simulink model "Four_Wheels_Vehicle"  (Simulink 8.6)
settings: Solver=ode45  StartTime=0.0  StopTime=20  RelTol=1e-3
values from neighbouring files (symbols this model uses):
  beta = 1    [Vehicle_Parameters.m]
  g = 9.81    [Vehicle_Parameters.m]
  H_CoG = 0.700    (= 0.7)    [Vehicle_Parameters.m]
  Hearo = 0.750    (= 0.75)    [Vehicle_Parameters.m]
  Iz = 2480    [Vehicle_Parameters.m]
  Jw = 2.166    [Vehicle_Parameters.m]
  L = 10    [Vehicle_Parameters.m]
  Lf = 1.180    (= 1.18)    [Vehicle_Parameters.m]
  Lr = 1.770    (= 1.77)    [Vehicle_Parameters.m]
  Lw = 1.880    (= 1.88)    [Vehicle_Parameters.m]
  m = 1500    [Vehicle_Parameters.m]
  miu = 0.85    [Vehicle_Parameters.m]
  reff = 0.380    (= 0.38)    [Vehicle_Parameters.m]
undefined symbols (not defined in the file or in its folder): DiscIntNeverNeededParam, Init, Ki, Kp, LowerLimit, sigbuilder_block, Ts, UpperLimit
libraries: simulink x15, powerlib_extras x3
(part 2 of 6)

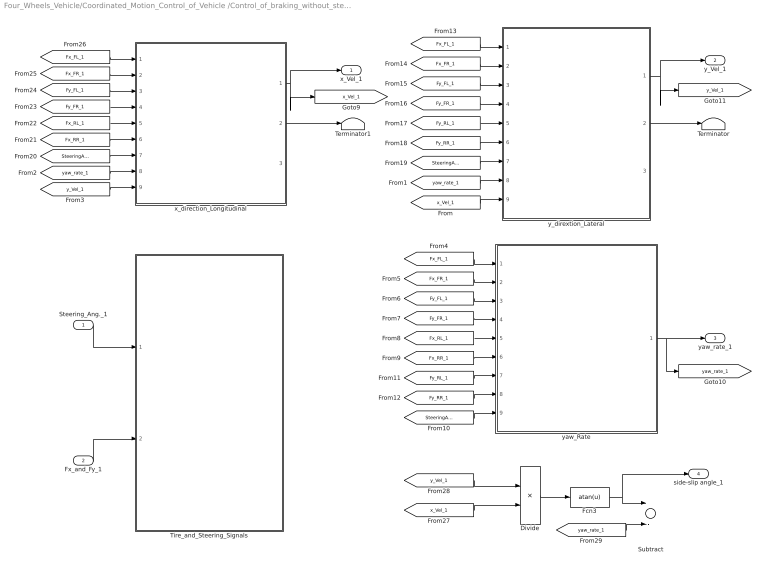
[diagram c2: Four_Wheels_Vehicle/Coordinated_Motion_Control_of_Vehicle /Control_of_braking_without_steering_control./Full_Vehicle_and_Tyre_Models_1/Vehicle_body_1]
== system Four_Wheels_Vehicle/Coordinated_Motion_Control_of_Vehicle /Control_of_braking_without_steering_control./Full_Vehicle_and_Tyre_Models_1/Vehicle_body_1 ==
  Steering_Ang._1 : Inport
  Fx_and_Fy_1 : Inport  Port=2
  Divide : Product  Inputs=*/
  Fcn3 : Fcn  Expr=atan(u)
  Subtract : Sum  Inputs=+-
  Terminator : Terminator
  Terminator1 : Terminator
  Tire_and_Steering_Signals : Subsystem
  x_direction_Longitudinal : Subsystem
  y_dirextion_Lateral : Subsystem
  yaw_Rate : Subsystem
  x_Vel_1 : Outport
  y_Vel_1 : Outport  Port=2
  yaw_rate_1 : Outport  Port=3
  side-slip angle_1 : Outport  Port=4
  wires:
  Fx_and_Fy_1/1 -> Tire_and_Steering_Signals/2(Fx_and_Fy)
  [yaw_rate_1] -> Subtract/2
  [y_Vel_1] -> Divide/1
  [x_Vel_1] -> Divide/2
  Fcn3/1 -> Subtract/1, side-slip angle_1/1
  Divide/1 -> Fcn3/1
  Steering_Ang._1/1 -> Tire_and_Steering_Signals/1(Steering_Ang.)
  yaw_Rate/1(yaw_rate_1) -> yaw_rate_1/1, [yaw_rate_1]
  [Fx_FL_1] -> x_direction_Longitudinal/1(Fx_FL_1)
  [Fx_FR_1] -> x_direction_Longitudinal/2(Fx_FR_1)
  [Fy_FL_1] -> x_direction_Longitudinal/3(Fy_FL_1)
  [Fy_FR_1] -> x_direction_Longitudinal/4(Fy_FR_1)
  [Fx_RL_1] -> x_direction_Longitudinal/5(Fx_RL_1)
  [Fx_RR_1] -> x_direction_Longitudinal/6(Fx_RR_1)
  [SteeringAng_1] -> x_direction_Longitudinal/7(Steering_Ang_1)
  [SteeringAng_1] -> y_dirextion_Lateral/7(Steering_Ang._1)
  [Fy_RR_1] -> y_dirextion_Lateral/6(Fy_RR_1)
  [Fy_RL_1] -> y_dirextion_Lateral/5(Fy_RL_1)
  [Fy_FR_1] -> y_dirextion_Lateral/4(Fy_FR_1)
  [Fy_FL_1] -> y_dirextion_Lateral/3(Fy_FL_1)
  [Fx_FR_1] -> y_dirextion_Lateral/2(Fx_FR_1)
  [Fx_FL_1] -> y_dirextion_Lateral/1(Fx_FL_1)
  [SteeringAng_1] -> yaw_Rate/9(Steering_Ang._1)
  [Fy_RR_1] -> yaw_Rate/8(Fy_RR_1)
  [Fy_RL_1] -> yaw_Rate/7(Fy_RL_1)
  [Fx_RR_1] -> yaw_Rate/6(Fx_RR_1)
  [Fx_RL_1] -> yaw_Rate/5(Fx_RL_1)
  [Fy_FR_1] -> yaw_Rate/4(Fy_FR_1)
  [Fy_FL_1] -> yaw_Rate/3(Fy_FL_1)
  [Fx_FR_1] -> yaw_Rate/2(Fx_FR_1)
  [Fx_FL_1] -> yaw_Rate/1(Fx_FL_1)
  [y_Vel_1] -> x_direction_Longitudinal/9(y_Vel_1)
  y_dirextion_Lateral/1(y_Vel_1) -> y_Vel_1/1, [y_Vel_1]
  [yaw_rate_1] -> x_direction_Longitudinal/8(yaw_rate_1)
  [yaw_rate_1] -> y_dirextion_Lateral/8(yaw_rate_1)
  [x_Vel_1] -> y_dirextion_Lateral/9(x_Vel_1)
  x_direction_Longitudinal/1(x_Vel_1) -> x_Vel_1/1, [x_Vel_1]
  x_direction_Longitudinal/2(x total force) -> Terminator1/1
  y_dirextion_Lateral/2(y total force) -> Terminator/1

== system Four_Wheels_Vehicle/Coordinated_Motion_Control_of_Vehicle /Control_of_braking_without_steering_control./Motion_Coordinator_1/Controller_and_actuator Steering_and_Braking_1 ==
  StteringAng : Inport
  Reference_Steering : Inport  Port=2
  Reference_Sideslip : Inport  Port=3
  Feedback_Steering : Inport  Port=4
  Feedback_Sideslip : Inport  Port=5
  Brake_controller_1 : Subsystem
  Brake_controller_2 : Subsystem
  Brake_controller_3 : Subsystem
  Brake_controller_4 : Subsystem
  Steering_controller : Subsystem
  f : Outport
  Mzc_1 : Outport  Port=2
  Mzc_2 : Outport  Port=3
  Mzc_3 : Outport  Port=4
  Mzc_4 : Outport  Port=5
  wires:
  Brake_controller_4/1(Mzc_4) -> Mzc_4/1
  Brake_controller_3/1(Mzc_3) -> Mzc_3/1
  Brake_controller_2/1(Mzc_2) -> Mzc_2/1
  Brake_controller_1/1(Mzc_1) -> Mzc_1/1
  Feedback_Sideslip/1 -> Brake_controller_1/2(Feedback_Sideslip_1), Brake_controller_2/2(Feedback_Sideslip_2), Brake_controller_3/2(Feedback_Sideslip_3), Brake_controller_4/2(Feedback_Sideslip_4)
  Reference_Sideslip/1 -> Brake_controller_1/1(Reference_Sideslip_1), Brake_controller_2/1(Reference_Sideslip_2), Brake_controller_3/1(Reference_Sideslip_3), Brake_controller_4/1(Reference_Sideslip_4)
  Steering_controller/1(f) -> f/1
  Feedback_Steering/1 -> Steering_controller/3(Feedback_Steering)
  Reference_Steering/1 -> Steering_controller/2(Reference_Steering)
  StteringAng/1 -> Steering_controller/1(StteringAng)

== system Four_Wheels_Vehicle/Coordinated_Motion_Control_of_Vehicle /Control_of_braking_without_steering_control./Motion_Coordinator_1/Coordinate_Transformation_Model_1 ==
  note: vehicle heading
  delta_steer (rad) : Inport
  v_x (m/s) : Inport  Port=2
  1/L : Gain  Gain=1/L
  Beta : Scope
  Beta1 : Scope
  Divide : Product  Inputs=*/
  Gain : Gain  Gain=L/2
  Gain1 : Gain  Gain=0.1
  Gain2 : Gain  Gain=0.1
  Gain4 : Gain  Gain=0.345
  Ground : Ground
  Integrator : Integrator
  Integrator1 : Integrator  LimitOutput=on  UpperSaturationLimit=0
  Integrator2 : Integrator
  Product{,1,3..4} (4 alike) : Product
  Sideslip_angle : Scope
  Subtract : Sum  Inputs=+-
  Sum : Sum  Inputs=|+-
  Sum1 : Sum  Inputs=|++
  Terminator : Terminator
  Trigonometric Function : Trigonometry  Operator=cos
  Trigonometric Function1 : Trigonometry
  Trigonometric Function2 : Trigonometry  Operator=atan
  Trigonometric Function3 : Trigonometry  Operator=tan
  steerVsYawrate1 : Scope  NumInputPorts=3
  steerVsYawrate2 : Scope  NumInputPorts=3
  yaw_rate : Product
  X-position : Outport
  Y-position : Outport  Port=2
  yaw_Rate : Outport  Port=3
  Sideslip_beta : Outport  Port=4
  yaw_pos. : Outport  Port=5
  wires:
  Subtract/1 -> Beta/1
  Gain4/1 -> Divide/1, Integrator1/1, steerVsYawrate2/3
  Trigonometric Function2/1 -> Subtract/1, Sideslip_beta/1, Sideslip_angle/1
  Gain2/1 -> Integrator2/1
  Gain1/1 -> Trigonometric Function1/1, yaw_pos./1, steerVsYawrate1/3, Trigonometric Function/1
  delta_steer (rad)/1 -> yaw_rate/2
  Divide/1 -> Trigonometric Function2/1
  Trigonometric Function3/1 -> Terminator/1
  Ground/1 -> Trigonometric Function3/1
  Product4/1 -> Sum1/2
  Product3/1 -> Sum/2
  Gain/1 -> Product4/1, Product3/1  "L/2*psi-dot"
  Sum1/1 -> Gain4/1  "v_Y (m/s)"
  Sum/1 -> Divide/2, Integrator/1, steerVsYawrate2/2  "v_X (m/s)"
  1/L/1 -> yaw_rate/1  "v_x / L"
  yaw_rate/1 -> Gain2/1, yaw_Rate/1, Subtract/2, Beta1/1, Gain/1, steerVsYawrate2/1
  v_x (m/s)/1 -> 1/L/1, Product1/1, Product/1  "v_x (m/s)"
  Integrator1/1 -> Y-position/1, steerVsYawrate1/2
  Integrator/1 -> X-position/1, steerVsYawrate1/1
  Integrator2/1 -> Gain1/1  "yaw_heading (rad)"
  Trigonometric Function1/1 -> Product3/2, Product/2  "sin(psi)"
  Trigonometric Function/1 -> Product4/2, Product1/2  "cos(psi)"
  Product1/1 -> Sum/1
  Product/1 -> Sum1/1

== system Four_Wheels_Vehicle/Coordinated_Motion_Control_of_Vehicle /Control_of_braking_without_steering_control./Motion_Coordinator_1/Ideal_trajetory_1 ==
  SteeringAng : Inport
  Constant_speed (m/s)1 : Constant  Value=4.55
  Coordinate_Transformation_Model : Subsystem
  Gain4 : Gain  Gain=10
  Y-position : Outport
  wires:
  SteeringAng/1 -> Gain4/1
  Constant_speed (m/s)1/1 -> Coordinate_Transformation_Model/2(v_x (m/s))
  Gain4/1 -> Coordinate_Transformation_Model/1(delta_steer (rad))
  Coordinate_Transformation_Model/2(Y-position) -> Y-position/1

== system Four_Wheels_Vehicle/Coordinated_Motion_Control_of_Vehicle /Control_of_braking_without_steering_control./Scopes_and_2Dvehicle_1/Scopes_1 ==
  SteeringAng_1 : Inport
  x_Vel_1 : Inport  Port=2
  y_Vel_1 : Inport  Port=3
  yaw_rate_1 : Inport  Port=4
  sideslipAng_1 : Inport  Port=5
  Ideal_1 : Inport  Port=6
  Integrator : Integrator  LimitOutput=on
  Integrator1 : Integrator  LimitOutput=on  UpperSaturationLimit=0
  Trajectory_Comparison : Scope  NumInputPorts=2
  steerVsYawrate : Scope  NumInputPorts=2
  x_y_directions : Scope  NumInputPorts=2
  x_y_yaw : Scope  NumInputPorts=4
  Ideal_trajectory_1 : Outport
  Estimated_trajectory_1 : Outport  Port=2
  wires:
  SteeringAng_1/1 -> steerVsYawrate/1
  sideslipAng_1/1 -> x_y_yaw/4
  yaw_rate_1/1 -> x_y_yaw/3, steerVsYawrate/2
  Integrator1/1 -> Trajectory_Comparison/2, Estimated_trajectory_1/1, x_y_directions/2
  Ideal_1/1 -> Ideal_trajectory_1/1, Trajectory_Comparison/1
  y_Vel_1/1 -> x_y_yaw/2, Integrator1/1
  x_Vel_1/1 -> x_y_yaw/1, Integrator/1
  Integrator/1 -> x_y_directions/1

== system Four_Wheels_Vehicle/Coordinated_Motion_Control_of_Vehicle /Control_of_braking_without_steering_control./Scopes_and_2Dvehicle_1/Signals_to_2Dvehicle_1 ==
  SteeringAng._1 : Inport
  x_Vel._1 : Inport  Port=2
  y_Vel._1 : Inport  Port=3
  yaw_rate._1 : Inport  Port=4
  Ideal._1 : Inport  Port=5
  Gain3 : Gain  Gain=0.05
  Integrator2 : Integrator  LimitOutput=on
  Integrator3 : Integrator  LimitOutput=on  UpperSaturationLimit=0
  Integrator4 : Integrator  LimitOutput=on  UpperSaturationLimit=0
  x_Vel_1 : Outport
  y_Vel_1 : Outport  Port=2
  yaw_rate_1 : Outport  Port=3
  SteeringAng_1 : Outport  Port=4
  Ideal_1 : Outport  Port=5
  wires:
  Ideal._1/1 -> Ideal_1/1
  SteeringAng._1/1 -> SteeringAng_1/1
  Gain3/1 -> yaw_rate_1/1
  Integrator3/1 -> y_Vel_1/1
  Integrator2/1 -> x_Vel_1/1
  yaw_rate._1/1 -> Integrator4/1
  Integrator4/1 -> Gain3/1
  y_Vel._1/1 -> Integrator3/1
  x_Vel._1/1 -> Integrator2/1

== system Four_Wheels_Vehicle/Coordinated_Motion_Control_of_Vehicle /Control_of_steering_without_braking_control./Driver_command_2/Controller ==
  Feedback : Inport
  Reference : Inport  Port=2
  Controller : powerlib_extras/Discrete  Control Blocks/Discrete PI Controller  Kp=20  Ki=0.15  Par_Limits=[10 -10]  Init=0  Ts=800e-6
  Scope3 : Scope
  Sum1 : Sum  Inputs=-+
  Td (N-m) : Outport
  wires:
  Feedback/1 -> Sum1/1
  Sum1/1 -> Controller/1
  Controller/1 -> Scope3/1, Td (N-m)/1
  Reference/1 -> Sum1/2

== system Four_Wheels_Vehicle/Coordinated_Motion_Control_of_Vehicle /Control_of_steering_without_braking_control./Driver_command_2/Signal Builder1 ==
  Demux : Demux  Tag=STV Demux  Outputs=2
  FromWs : FromWorkspace  Tag=STV FromWs  VariableName=tuvar  SampleTime=0  SigBuilderData=DataTag6  VnvData=DataTag7
  Signal 1 : Outport  Tag=STV Outport
  Signal 2 : Outport  Tag=STV Outport  Port=2
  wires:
  Demux/2 -> Signal 2/1
  FromWs/1 -> Demux/1
  Demux/1 -> Signal 1/1

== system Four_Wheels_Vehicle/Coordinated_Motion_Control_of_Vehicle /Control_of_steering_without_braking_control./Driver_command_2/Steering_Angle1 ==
  Demux : Demux  Tag=STV Demux  Outputs=2
  FromWs : FromWorkspace  Tag=STV FromWs  VariableName=tuvar  SampleTime=0  SigBuilderData=DataTag8  VnvData=DataTag9
  Imported_Signal 1 : Outport  Tag=STV Outport
  Signal 1 : Outport  Tag=STV Outport  Port=2
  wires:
  FromWs/1 -> Demux/1
  Demux/1 -> Imported_Signal 1/1
  Demux/2 -> Signal 1/1

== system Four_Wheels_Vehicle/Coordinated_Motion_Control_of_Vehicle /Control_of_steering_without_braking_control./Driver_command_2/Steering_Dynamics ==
  Driver Torque : Inport
  Add : Sum  Inputs=+---
  Gain : Gain  Gain=25
  Gain1 : Gain  Gain=0.0065
  Gain2 : Gain  Gain=360/(2*pi)
  Gain3 : Gain  Gain=115
  Gain5 : Gain  Gain=2
  Gain6 : Gain  Gain=0.361
  Integrator : Integrator
  Integrator1 : Integrator
  Saturation : Saturate  UpperLimit=1  LowerLimit=-1
  Scope{1..5,8,10} (7 alike) : Scope
  Sign1 : Signum
  Steering Wheel Angle : Outport
  Ts : Outport  Port=2
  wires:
  Integrator1/1 -> Sign1/1, Saturation/1, Gain3/1, Gain2/1
  Gain/1 -> Scope8/1, Integrator/1
  Add/1 -> Gain/1
  Driver Torque/1 -> Scope10/1, Add/1
  Gain2/1 -> Scope2/1, Steering Wheel Angle/1
  Gain3/1 -> Ts/1, Add/2, Scope1/1
  Gain5/1 -> Add/4, Scope5/1
  Gain1/1 -> Scope3/1, Add/3
  Gain6/1 -> Gain5/1
  Integrator/1 -> Integrator1/1, Gain6/1, Scope4/1
  Saturation/1 -> Gain1/1

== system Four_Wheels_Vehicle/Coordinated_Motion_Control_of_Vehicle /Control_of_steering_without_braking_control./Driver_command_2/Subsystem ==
  Product : Product
  Ramp : simulink/Sources/Ramp  slope=3  start=0  X0=0
  Scope : Scope
  Scope1 : Scope
  Trigonometric Function : Trigonometry
  Steering_Ang. : Outport
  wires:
  Ramp/1 -> Product/1, Trigonometric Function/1
  Trigonometric Function/1 -> Product/2, Scope/1
  Product/1 -> Steering_Ang./1, Scope1/1

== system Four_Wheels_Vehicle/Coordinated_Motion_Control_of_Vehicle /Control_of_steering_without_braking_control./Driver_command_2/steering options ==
  (+) bias --> RH turn (-) bias --> LH turn1 : Constant  Value=0.5
  (+) bias --> RH turn (-) bias --> LH turn2 : Constant  Value=0.5
  Display{,1..3} (4 alike) : Display
  Gain : Gain  Gain=0.5
  Gain1 : Gain  Gain=-0.5
  Gain{2..5} (4 alike) : Gain
  Multiport Switch : MultiPortSwitch
  Sum{,1..3} (4 alike) : Sum  Inputs=|++
  left turn? : ManualSwitch  CurrentSetting=0
  restart point for: data received average1 : Constant
  restart point for: data received average2 : Constant  Value=0
  restart point for: data received average3 : Constant
  restart point for: data received average4 : Constant  Value=0
  right turn? : ManualSwitch  CurrentSetting=0
  steer select : Constant  Value=3
  turn LEFT hard : Step  Time=10  After=-1  SampleTime=0
  turn LEFT medium : Step  Time=30  After=-0.5  SampleTime=0
  turn RIGHT hard : Step  Time=20  After=+1  SampleTime=0
  delta_steer (rad) : Outport
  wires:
  (+) bias --> RH turn (-) bias --> LH turn2/1 -> Multiport Switch/2  "delta_steer (rad)"
  steer select/1 -> Multiport Switch/1
  Multiport Switch/1 -> delta_steer (rad)/1
  restart point for: data received average1/1 -> right turn?/1
  restart point for: data received average2/1 -> right turn?/2
  Sum/1 -> Multiport Switch/3
  right turn?/1 -> Gain/1
  restart point for: data received average3/1 -> left turn?/1
  restart point for: data received average4/1 -> left turn?/2
  left turn?/1 -> Gain1/1
  Gain/1 -> Sum/1
  Gain1/1 -> Sum/2
  Sum1/1 -> Multiport Switch/4, Display/1
  (+) bias --> RH turn (-) bias --> LH turn1/1 -> Gain5/1
  turn RIGHT hard/1 -> Gain3/1
  turn LEFT medium/1 -> Gain4/1
  turn LEFT hard/1 -> Gain2/1
  Sum2/1 -> Display2/1, Sum3/2
  Sum3/1 -> Display3/1, Sum1/2
  Gain2/1 -> Sum3/1
  Gain3/1 -> Sum2/1
  Gain4/1 -> Display1/1, Sum2/2
  Gain5/1 -> Sum1/1

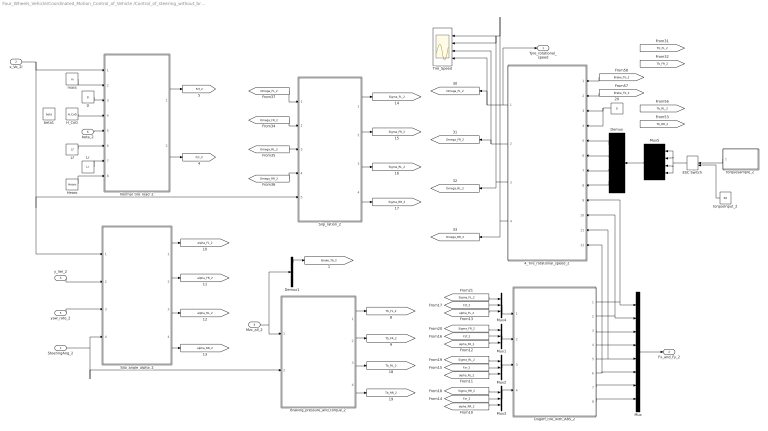
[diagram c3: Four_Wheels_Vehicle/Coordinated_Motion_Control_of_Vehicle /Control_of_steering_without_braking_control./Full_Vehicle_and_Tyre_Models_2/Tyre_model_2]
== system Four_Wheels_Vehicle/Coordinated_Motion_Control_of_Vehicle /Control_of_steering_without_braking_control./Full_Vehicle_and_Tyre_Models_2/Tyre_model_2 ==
  SteeringAng_2 : Inport
  x_Ve_2l : Inport  Port=2
  y_Vel_2 : Inport  Port=3
  Mzc_all_2 : Inport  Port=4
  yaw_rate_2 : Inport  Port=5
  beta_2 : Inport  Port=6
  20 : Constant  Value=0
  4_Tire_rotational_speed_2 : Subsystem
  Braking_pressure_and_torque_2 : Subsystem
  Demux : Demux
  Demux1 : Demux
  Dugoff_tire_with_ABS_2 : Subsystem
  ESC Switch : ManualSwitch
  H_CoG : Constant  Value=H_CoG
  Hearo : Constant  Value=Hearo
  Lf : Constant  Value=Lf
  Lr : Constant  Value=Lr
  Mux : Mux  Inputs=8
  Mux{1..4} (4 alike) : Mux  Inputs=3
  Mux5 : Mux
  Normal_tire_load_2 : Subsystem
  Slip_angle_alpha_2 : Subsystem
  Slip_ration_2 : Subsystem
  Tire_Speed : Scope  NumInputPorts=4
  beta1 : Constant  Value=beta
  g : Constant  Value=g
  mass : Constant  Value=m
  torqueInput_2 : Constant  Value=50
  "torquesample_2 " : Subsystem  Tag=STV Subsys  LoadFcn=sigbuilder_block('load');  StartFcn=sigbuilder_block('start');  StopFcn=sigbuilder_block('stop');  ClipboardFcn=sigbuilder_block('clipboard');
  Tyre_rotational_speed : Outport
  Fx_and_Fy_2 : Outport  Port=2
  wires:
  Braking_pressure_and_torque_2/4(Tb_RR_2) -> [Tb_RR_2]
  Mzc_all_2/1 -> Demux1/1, Braking_pressure_and_torque_2/1(Mzc_all_2)
  Braking_pressure_and_torque_2/1(Tb_FL_2) -> [Tb_FL_2]
  Braking_pressure_and_torque_2/2(Tb_FR_2) -> [Tb_FR_2]
  Braking_pressure_and_torque_2/3(Tb_RL_2) -> [Tb_RL_2]
  yaw_rate_2/1 -> Slip_angle_alpha_2/3(yaw_rate_2)
  Slip_ration_2/4(Sigma_RR_2) -> [Sigma_RR_2]
  [alpha_RL_2] -> Mux2/3
  Mux2/1 -> Dugoff_tire_with_ABS_2/3(In5)
  y_Vel_2/1 -> Slip_angle_alpha_2/2(y_Vel_2)
  Slip_ration_2/3(Sigma_RL_2) -> [Sigma_RL_2]
  Slip_ration_2/1(Sigma_FL_2) -> [Sigma_FL_2]
  Mux3/1 -> Dugoff_tire_with_ABS_2/4(In3)
  Mux1/1 -> Dugoff_tire_with_ABS_2/2(In2)
  Mux4/1 -> Dugoff_tire_with_ABS_2/1(In1)
  [alpha_RR_2] -> Mux3/3
  Slip_ration_2/2(Sigma_FR_2) -> [Sigma_FR_2]
  Lr/1 -> Normal_tire_load_2/7(Lr)
  4_Tire_rotational_speed_2/1(Omega_FL_2) -> Tyre_rotational_speed/1, Tire_Speed/4, [Omega_FL_2]
  Demux/2 -> 4_Tire_rotational_speed_2/6(Td_FR_2)
  "torquesample_2 "/1(Signal 1) -> ESC Switch/1
  Dugoff_tire_with_ABS_2/5(Fx_RL_2) -> Mux/5, 4_Tire_rotational_speed_2/11(Fx_RL_2)
  SteeringAng_2/1 -> Braking_pressure_and_torque_2/2(SteeringAng), Slip_angle_alpha_2/4(Steering_Ang._2)
  [Sigma_RL_2] -> Mux2/1
  Lf/1 -> Normal_tire_load_2/6(Lf)
  H_CoG/1 -> Normal_tire_load_2/4(H_CoG)
  4_Tire_rotational_speed_2/3(Omega_RL_2) -> Tire_Speed/2, [Omega_RL_2]
  Mux5/1 -> Demux/1
  ESC Switch/1 -> Mux5/4, Mux5/3, Mux5/1, Mux5/2
  [Omega_FR_2] -> Slip_ration_2/2(Omega_FR_2)
  Demux/3 -> 4_Tire_rotational_speed_2/7(Td_RL_2)
  [alpha_FR_2] -> Mux1/3
  Dugoff_tire_with_ABS_2/6(Fx_RR_2) -> Mux/6, 4_Tire_rotational_speed_2/12(Fx_RR_2)
  [alpha_FL_2] -> Mux4/3
  Demux/4 -> 4_Tire_rotational_speed_2/8(Td_RR_2)
  [Omega_FL_2] -> Slip_ration_2/1(Omega_FL_2)
  [Omega_RR_2] -> Slip_ration_2/4(Omega_RR_2)
  [Sigma_FR_2] -> Mux1/1
  x_Ve_2l/1 -> Slip_angle_alpha_2/1(x_Vel_2), Slip_ration_2/5(x_Vel_2), Normal_tire_load_2/1(x_Vel_2)
  [Omega_RL_2] -> Slip_ration_2/3(Omega_RL_2)
  Dugoff_tire_with_ABS_2/2(Fx_FR_2) -> Mux/2, 4_Tire_rotational_speed_2/10(Fx_FR_2)
  [Sigma_RR_2] -> Mux3/1
  Dugoff_tire_with_ABS_2/1(Fx_FL_2) -> Mux/1, 4_Tire_rotational_speed_2/9(Fx_FL_2)
  beta_2/1 -> Normal_tire_load_2/5(beta)
  mass/1 -> Normal_tire_load_2/2(mass)
  [Sigma_FL_2] -> Mux4/1
  4_Tire_rotational_speed_2/2(Omega_FR_2) -> Tire_Speed/3, [Omega_FR_2]
  Normal_tire_load_2/2(Fz_r_2) -> [Fzr_2]
  Hearo/1 -> Normal_tire_load_2/8(Hearo)
  g/1 -> Normal_tire_load_2/3(g)
  Demux/1 -> 4_Tire_rotational_speed_2/5(Td_FL_2)
  torqueInput_2/1 -> ESC Switch/2
  Slip_angle_alpha_2/4(alpha_RR_2) -> [alpha_RR_2]
  [Fzf_2] -> Mux4/2
  20/1 -> 4_Tire_rotational_speed_2/4(Tb_RR_2), 4_Tire_rotational_speed_2/3(Tb_RL_2)
  4_Tire_rotational_speed_2/4(Omega_RR_2) -> Tire_Speed/1, [Omega_RR_2]
  [Fzr_2] -> Mux3/2
  [Brake_Tb_2] -> 4_Tire_rotational_speed_2/1(Tb_FL_2)
  [Brake_Tb_2] -> 4_Tire_rotational_speed_2/2(Tb_FR_2)
  Normal_tire_load_2/1(Fz_f_2) -> [Fzf_2]
  [Fzr_2] -> Mux2/2
  [Fzf_2] -> Mux1/2
  Slip_angle_alpha_2/3(alpha_RL_2) -> [alpha_RL_2]
  Slip_angle_alpha_2/1(alpha_FL_2) -> [alpha_FL_2]
  Slip_angle_alpha_2/2(alpha_FR_2) -> [alpha_FR_2]
  Dugoff_tire_with_ABS_2/8(Fy_RR_2) -> Mux/8
  Dugoff_tire_with_ABS_2/7(Fy_RL_2) -> Mux/7
  Dugoff_tire_with_ABS_2/4(Fy_FR_2) -> Mux/4
  Dugoff_tire_with_ABS_2/3(Fy_FL_2) -> Mux/3
  Mux/1 -> Fx_and_Fy_2/1
  Demux1/1 -> [Brake_Tb_2]

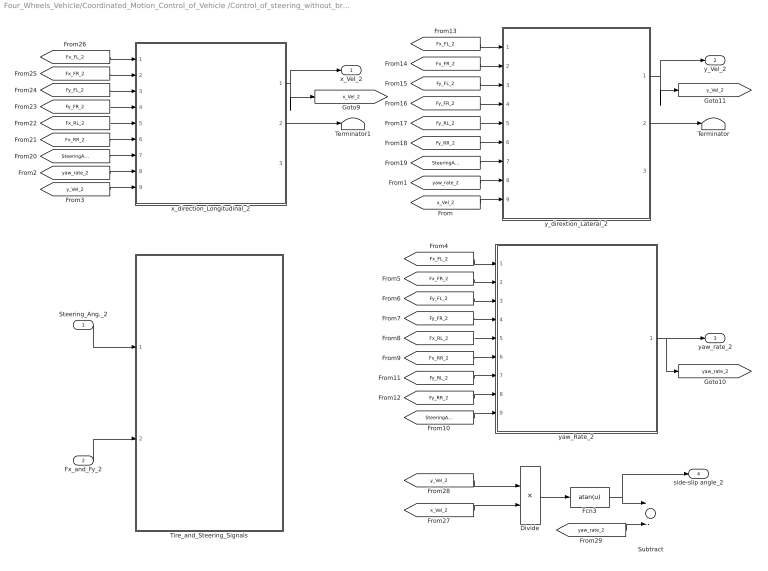
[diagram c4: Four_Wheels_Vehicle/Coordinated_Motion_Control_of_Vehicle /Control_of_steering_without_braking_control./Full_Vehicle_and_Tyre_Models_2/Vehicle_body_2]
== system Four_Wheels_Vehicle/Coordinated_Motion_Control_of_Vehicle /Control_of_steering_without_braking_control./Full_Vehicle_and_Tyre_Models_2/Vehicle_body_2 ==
  Steering_Ang._2 : Inport
  Fx_and_Fy_2 : Inport  Port=2
  Divide : Product  Inputs=*/
  Fcn3 : Fcn  Expr=atan(u)
  Subtract : Sum  Inputs=+-
  Terminator : Terminator
  Terminator1 : Terminator
  Tire_and_Steering_Signals : Subsystem
  x_direction_Longitudinal_2 : Subsystem
  y_dirextion_Lateral_2 : Subsystem
  yaw_Rate_2 : Subsystem
  x_Vel_2 : Outport
  y_Vel_2 : Outport  Port=2
  yaw_rate_2 : Outport  Port=3
  side-slip angle_2 : Outport  Port=4
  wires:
  y_dirextion_Lateral_2/2(y total force) -> Terminator/1
  x_direction_Longitudinal_2/2(x total force) -> Terminator1/1
  x_direction_Longitudinal_2/1(x_Vel_2) -> [x_Vel_2], x_Vel_2/1
  [x_Vel_2] -> y_dirextion_Lateral_2/9(x_Vel_2)
  [yaw_rate_2] -> y_dirextion_Lateral_2/8(yaw_rate_2)
  [yaw_rate_2] -> x_direction_Longitudinal_2/8(yaw_rate_2)
  y_dirextion_Lateral_2/1(y_Vel_2) -> [y_Vel_2], y_Vel_2/1
  [y_Vel_2] -> x_direction_Longitudinal_2/9(y_Vel_2)
  [Fx_FL_2] -> yaw_Rate_2/1(Fx_FL_2)
  [Fx_FR_2] -> yaw_Rate_2/2(Fx_FR_2)
  [Fy_FL_2] -> yaw_Rate_2/3(Fy_FL_2)
  [Fy_FR_2] -> yaw_Rate_2/4(Fy_FR_2)
  [Fx_RL_2] -> yaw_Rate_2/5(Fx_RL_2)
  [Fx_RR_2] -> yaw_Rate_2/6(Fx_RR_2)
  [Fy_RL_2] -> yaw_Rate_2/7(Fy_RL_2)
  [Fy_RR_2] -> yaw_Rate_2/8(Fy_RR_2)
  [SteeringAng_2] -> yaw_Rate_2/9(Steering_Ang._2)
  [Fx_FL_2] -> y_dirextion_Lateral_2/1(Fx_FL_2)
  [Fx_FR_2] -> y_dirextion_Lateral_2/2(Fx_FR_2)
  [Fy_FL_2] -> y_dirextion_Lateral_2/3(Fy_FL_2)
  [Fy_FR_2] -> y_dirextion_Lateral_2/4(Fy_FR_2)
  [Fy_RL_2] -> y_dirextion_Lateral_2/5(Fy_RL_2)
  [Fy_RR_2] -> y_dirextion_Lateral_2/6(Fy_RR_2)
  [SteeringAng_2] -> y_dirextion_Lateral_2/7(Steering_Ang._2)
  [SteeringAng_2] -> x_direction_Longitudinal_2/7(Steering_Ang._2)
  [Fx_RR_2] -> x_direction_Longitudinal_2/6(Fx_RR_2)
  [Fx_RL_2] -> x_direction_Longitudinal_2/5(Fx_RL_2)
  [Fy_FR_2] -> x_direction_Longitudinal_2/4(Fy_FR_2)
  [Fy_FL_2] -> x_direction_Longitudinal_2/3(Fy_FL_2)
  [Fx_FR_2] -> x_direction_Longitudinal_2/2(Fx_FR_2)
  [Fx_FL_2] -> x_direction_Longitudinal_2/1(Fx_FL_2)
  yaw_Rate_2/1(yaw_rate_2) -> [yaw_rate_2], yaw_rate_2/1
  Steering_Ang._2/1 -> Tire_and_Steering_Signals/1(Steering_Ang._2)
  Divide/1 -> Fcn3/1
  Fcn3/1 -> side-slip angle_2/1, Subtract/1
  [x_Vel_2] -> Divide/2
  [y_Vel_2] -> Divide/1
  [yaw_rate_2] -> Subtract/2
  Fx_and_Fy_2/1 -> Tire_and_Steering_Signals/2(Fx_and_Fy_2)

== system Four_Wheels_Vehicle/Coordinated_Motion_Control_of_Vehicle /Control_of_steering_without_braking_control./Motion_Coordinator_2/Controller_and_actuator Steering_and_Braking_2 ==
  StteringAng : Inport
  Reference_Steering : Inport  Port=2
  Reference_Sideslip : Inport  Port=3
  Feedback_Steering : Inport  Port=4
  Feedback_Sideslip : Inport  Port=5
  Brake_controller_1 : Subsystem
  Brake_controller_2 : Subsystem
  Brake_controller_3 : Subsystem
  Brake_controller_4 : Subsystem
  Steering_controller : Subsystem
  f : Outport
  Mzc_1 : Outport  Port=2
  Mzc_2 : Outport  Port=3
  Mzc_3 : Outport  Port=4
  Mzc_4 : Outport  Port=5
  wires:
  StteringAng/1 -> Steering_controller/1(StteringAng)
  Reference_Steering/1 -> Steering_controller/2(Reference_Steering)
  Feedback_Steering/1 -> Steering_controller/3(Feedback_Steering)
  Steering_controller/1(f) -> f/1
  Reference_Sideslip/1 -> Brake_controller_4/1(Reference_Sideslip_4), Brake_controller_3/1(Reference_Sideslip_3), Brake_controller_2/1(Reference_Sideslip_2), Brake_controller_1/1(Reference_Sideslip_1)
  Feedback_Sideslip/1 -> Brake_controller_4/2(Feedback_Sideslip_4), Brake_controller_3/2(Feedback_Sideslip_3), Brake_controller_2/2(Feedback_Sideslip_2), Brake_controller_1/2(Feedback_Sideslip_1)
  Brake_controller_1/1(Mzc_1) -> Mzc_1/1
  Brake_controller_2/1(Mzc_2) -> Mzc_2/1
  Brake_controller_3/1(Mzc_3) -> Mzc_3/1
  Brake_controller_4/1(Mzc_4) -> Mzc_4/1

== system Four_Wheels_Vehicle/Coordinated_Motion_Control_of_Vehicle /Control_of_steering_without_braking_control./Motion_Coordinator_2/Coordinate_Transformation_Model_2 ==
  note: vehicle heading
  delta_steer (rad) : Inport
  v_x (m/s) : Inport  Port=2
  1/L : Gain  Gain=1/L
  Beta : Scope
  Beta1 : Scope
  Divide : Product  Inputs=*/
  Gain : Gain  Gain=L/2
  Gain1 : Gain  Gain=0.1
  Gain2 : Gain  Gain=0.1
  Gain4 : Gain  Gain=0.345
  Ground : Ground
  Integrator : Integrator
  Integrator1 : Integrator  LimitOutput=on  UpperSaturationLimit=0
  Integrator2 : Integrator
  Product{,1,3..4} (4 alike) : Product
  Sideslip_angle : Scope
  Subtract : Sum  Inputs=+-
  Sum : Sum  Inputs=|+-
  Sum1 : Sum  Inputs=|++
  Terminator : Terminator
  Trigonometric Function : Trigonometry  Operator=cos
  Trigonometric Function1 : Trigonometry
  Trigonometric Function2 : Trigonometry  Operator=atan
  Trigonometric Function3 : Trigonometry  Operator=tan
  steerVsYawrate1 : Scope  NumInputPorts=3
  steerVsYawrate2 : Scope  NumInputPorts=3
  yaw_rate : Product
  X-position : Outport
  Y-position : Outport  Port=2
  yaw_Rate : Outport  Port=3
  Sideslip_beta : Outport  Port=4
  yaw_pos._2 : Outport  Port=5
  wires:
  Product/1 -> Sum1/1
  Product1/1 -> Sum/1
  Trigonometric Function/1 -> Product1/2, Product4/2  "cos(psi)"
  Trigonometric Function1/1 -> Product/2, Product3/2  "sin(psi)"
  Integrator2/1 -> Gain1/1  "yaw_heading (rad)"
  Integrator/1 -> steerVsYawrate1/1, X-position/1
  Integrator1/1 -> steerVsYawrate1/2, Y-position/1
  v_x (m/s)/1 -> Product/1, Product1/1, 1/L/1  "v_x (m/s)"
  yaw_rate/1 -> steerVsYawrate2/1, Gain/1, Beta1/1, Subtract/2, yaw_Rate/1, Gain2/1
  1/L/1 -> yaw_rate/1  "v_x / L"
  Sum/1 -> steerVsYawrate2/2, Integrator/1, Divide/2  "v_X (m/s)"
  Sum1/1 -> Gain4/1  "v_Y (m/s)"
  Gain/1 -> Product3/1, Product4/1  "L/2*psi-dot"
  Product3/1 -> Sum/2
  Product4/1 -> Sum1/2
  Ground/1 -> Trigonometric Function3/1
  Trigonometric Function3/1 -> Terminator/1
  Divide/1 -> Trigonometric Function2/1
  delta_steer (rad)/1 -> yaw_rate/2
  Gain1/1 -> Trigonometric Function/1, yaw_pos._2/1, steerVsYawrate1/3, Trigonometric Function1/1
  Gain2/1 -> Integrator2/1
  Trigonometric Function2/1 -> Sideslip_angle/1, Sideslip_beta/1, Subtract/1
  Gain4/1 -> steerVsYawrate2/3, Integrator1/1, Divide/1
  Subtract/1 -> Beta/1

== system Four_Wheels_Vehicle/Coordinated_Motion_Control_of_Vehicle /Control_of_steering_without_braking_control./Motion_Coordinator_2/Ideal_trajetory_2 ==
  SteeringAng : Inport
  Constant_speed (m/s)1 : Constant  Value=4.55
  Coordinate_Transformation_Model : Subsystem
  Gain4 : Gain  Gain=10
  Y-position : Outport
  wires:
  Coordinate_Transformation_Model/2(Y-position) -> Y-position/1
  Gain4/1 -> Coordinate_Transformation_Model/1(delta_steer (rad))
  Constant_speed (m/s)1/1 -> Coordinate_Transformation_Model/2(v_x (m/s))
  SteeringAng/1 -> Gain4/1

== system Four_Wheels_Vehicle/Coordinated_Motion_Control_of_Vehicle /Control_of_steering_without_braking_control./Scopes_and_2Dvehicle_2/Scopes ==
  SteeringAng_2 : Inport
  x_Vel_2 : Inport  Port=2
  y_Vel_2 : Inport  Port=3
  yaw_rate_2 : Inport  Port=4
  sideslipAng_2 : Inport  Port=5
  Ideal_2 : Inport  Port=6
  Integrator : Integrator  LimitOutput=on
  Integrator1 : Integrator  LimitOutput=on  UpperSaturationLimit=0
  Trajectory_Comparison : Scope  NumInputPorts=2
  steerVsYawrate : Scope  NumInputPorts=2
  x_y_directions : Scope  NumInputPorts=2
  x_y_yaw : Scope  NumInputPorts=4
  Ideal_trajectory_2 : Outport
  Estimated_trajectory_2 : Outport  Port=2
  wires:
  Integrator/1 -> x_y_directions/1
  x_Vel_2/1 -> Integrator/1, x_y_yaw/1
  y_Vel_2/1 -> Integrator1/1, x_y_yaw/2
  Ideal_2/1 -> Trajectory_Comparison/1, Ideal_trajectory_2/1
  Integrator1/1 -> x_y_directions/2, Estimated_trajectory_2/1, Trajectory_Comparison/2
  yaw_rate_2/1 -> steerVsYawrate/2, x_y_yaw/3
  sideslipAng_2/1 -> x_y_yaw/4
  SteeringAng_2/1 -> steerVsYawrate/1

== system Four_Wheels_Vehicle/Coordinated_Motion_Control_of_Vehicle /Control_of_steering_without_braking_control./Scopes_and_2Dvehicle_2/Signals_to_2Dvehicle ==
  SteeringAng._2 : Inport
  x_Vel._2 : Inport  Port=2
  y_Vel._2 : Inport  Port=3
  yaw_rate._2 : Inport  Port=4
  Ideal._2 : Inport  Port=5
  Gain1 : Gain  Gain=0.95
  Gain3 : Gain  Gain=0.05
  Integrator2 : Integrator  LimitOutput=on
  Integrator3 : Integrator  LimitOutput=on  UpperSaturationLimit=0
  Integrator4 : Integrator  LimitOutput=on  UpperSaturationLimit=0
  x_Vel_2 : Outport
  y_Vel_2 : Outport  Port=2
  yaw_rate_2 : Outport  Port=3
  SteeringAng_2 : Outport  Port=4
  Ideal_2 : Outport  Port=5
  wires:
  x_Vel._2/1 -> Integrator2/1
  y_Vel._2/1 -> Integrator3/1
  Integrator4/1 -> Gain3/1
  yaw_rate._2/1 -> Integrator4/1
  Integrator2/1 -> x_Vel_2/1
  Integrator3/1 -> Gain1/1
  Gain3/1 -> yaw_rate_2/1
  SteeringAng._2/1 -> SteeringAng_2/1
  Ideal._2/1 -> Ideal_2/1
  Gain1/1 -> y_Vel_2/1

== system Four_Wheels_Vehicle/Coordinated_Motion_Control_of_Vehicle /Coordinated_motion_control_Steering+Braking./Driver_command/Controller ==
  Feedback : Inport
  Reference : Inport  Port=2
  Controller : powerlib_extras/Discrete  Control Blocks/Discrete PI Controller  Kp=20  Ki=0.15  Par_Limits=[10 -10]  Init=0  Ts=800e-6
  Scope3 : Scope
  Sum1 : Sum  Inputs=-+
  Td (N-m) : Outport
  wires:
  Feedback/1 -> Sum1/1
  Sum1/1 -> Controller/1
  Controller/1 -> Scope3/1, Td (N-m)/1
  Reference/1 -> Sum1/2

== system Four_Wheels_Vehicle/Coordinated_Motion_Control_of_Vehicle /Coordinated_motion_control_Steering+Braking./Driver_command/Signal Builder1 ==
  Demux : Demux  Tag=STV Demux  Outputs=2
  FromWs : FromWorkspace  Tag=STV FromWs  VariableName=tuvar  SampleTime=0  SigBuilderData=DataTag12  VnvData=DataTag13
  Signal 1 : Outport  Tag=STV Outport
  Signal 2 : Outport  Tag=STV Outport  Port=2
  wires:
  Demux/2 -> Signal 2/1
  FromWs/1 -> Demux/1
  Demux/1 -> Signal 1/1

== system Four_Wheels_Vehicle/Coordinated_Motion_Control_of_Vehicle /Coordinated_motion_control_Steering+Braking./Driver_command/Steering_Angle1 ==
  Demux : Demux  Tag=STV Demux  Outputs=2
  FromWs : FromWorkspace  Tag=STV FromWs  VariableName=tuvar  SampleTime=0  SigBuilderData=DataTag14  VnvData=DataTag15
  Imported_Signal 1 : Outport  Tag=STV Outport
  Signal 1 : Outport  Tag=STV Outport  Port=2
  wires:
  FromWs/1 -> Demux/1
  Demux/1 -> Imported_Signal 1/1
  Demux/2 -> Signal 1/1

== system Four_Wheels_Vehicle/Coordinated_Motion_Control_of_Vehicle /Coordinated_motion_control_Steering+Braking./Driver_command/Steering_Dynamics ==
  Driver Torque : Inport
  Add : Sum  Inputs=+---
  Gain : Gain  Gain=25
  Gain1 : Gain  Gain=0.0065
  Gain2 : Gain  Gain=360/(2*pi)
  Gain3 : Gain  Gain=115
  Gain5 : Gain  Gain=2
  Gain6 : Gain  Gain=0.361
  Integrator : Integrator
  Integrator1 : Integrator
  Scope{1..5,8,10} (7 alike) : Scope
  Sign1 : Signum
  Transport Delay : TransportDelay  DelayTime=0.25
  Steering Wheel Angle : Outport
  Ts : Outport  Port=2
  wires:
  Gain/1 -> Scope8/1, Integrator/1
  Add/1 -> Gain/1
  Driver Torque/1 -> Scope10/1, Add/1
  Gain2/1 -> Scope2/1, Steering Wheel Angle/1
  Gain3/1 -> Ts/1, Add/2, Scope1/1
  Gain5/1 -> Add/4, Scope5/1
  Gain1/1 -> Scope3/1, Add/3
  Gain6/1 -> Gain5/1
  Integrator/1 -> Integrator1/1, Gain6/1, Scope4/1
  Integrator1/1 -> Gain1/1, Sign1/1, Transport Delay/1, Gain2/1
  Transport Delay/1 -> Gain3/1

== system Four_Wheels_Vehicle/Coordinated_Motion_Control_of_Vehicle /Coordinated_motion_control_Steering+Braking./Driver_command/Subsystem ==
  Product : Product
  Ramp : simulink/Sources/Ramp  slope=3  start=0  X0=0
  Scope : Scope
  Scope1 : Scope
  Trigonometric Function : Trigonometry
  Steering_Ang. : Outport
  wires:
  Ramp/1 -> Product/1, Trigonometric Function/1
  Trigonometric Function/1 -> Product/2, Scope/1
  Product/1 -> Steering_Ang./1, Scope1/1

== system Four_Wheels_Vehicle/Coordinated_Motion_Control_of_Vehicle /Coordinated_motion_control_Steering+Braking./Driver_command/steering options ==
  (+) bias --> RH turn (-) bias --> LH turn1 : Constant  Value=0.5
  (+) bias --> RH turn (-) bias --> LH turn2 : Constant  Value=0.5
  Display{,1..3} (4 alike) : Display
  Gain : Gain  Gain=0.5
  Gain1 : Gain  Gain=-0.5
  Gain{2..5} (4 alike) : Gain
  Multiport Switch : MultiPortSwitch
  Sum{,1..3} (4 alike) : Sum  Inputs=|++
  left turn? : ManualSwitch  CurrentSetting=0
  restart point for: data received average1 : Constant
  restart point for: data received average2 : Constant  Value=0
  restart point for: data received average3 : Constant
  restart point for: data received average4 : Constant  Value=0
  right turn? : ManualSwitch  CurrentSetting=0
  steer select : Constant  Value=3
  turn LEFT hard : Step  Time=10  After=-1  SampleTime=0
  turn LEFT medium : Step  Time=30  After=-0.5  SampleTime=0
  turn RIGHT hard : Step  Time=20  After=+1  SampleTime=0
  delta_steer (rad) : Outport
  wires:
  (+) bias --> RH turn (-) bias --> LH turn2/1 -> Multiport Switch/2  "delta_steer (rad)"
  steer select/1 -> Multiport Switch/1
  Multiport Switch/1 -> delta_steer (rad)/1
  restart point for: data received average1/1 -> right turn?/1
  restart point for: data received average2/1 -> right turn?/2
  Sum/1 -> Multiport Switch/3
  right turn?/1 -> Gain/1
  restart point for: data received average3/1 -> left turn?/1
  restart point for: data received average4/1 -> left turn?/2
  left turn?/1 -> Gain1/1
  Gain/1 -> Sum/1
  Gain1/1 -> Sum/2
  Sum1/1 -> Multiport Switch/4, Display/1
  (+) bias --> RH turn (-) bias --> LH turn1/1 -> Gain5/1
  turn RIGHT hard/1 -> Gain3/1
  turn LEFT medium/1 -> Gain4/1
  turn LEFT hard/1 -> Gain2/1
  Sum2/1 -> Display2/1, Sum3/2
  Sum3/1 -> Display3/1, Sum1/2
  Gain2/1 -> Sum3/1
  Gain3/1 -> Sum2/1
  Gain4/1 -> Display1/1, Sum2/2
  Gain5/1 -> Sum1/1

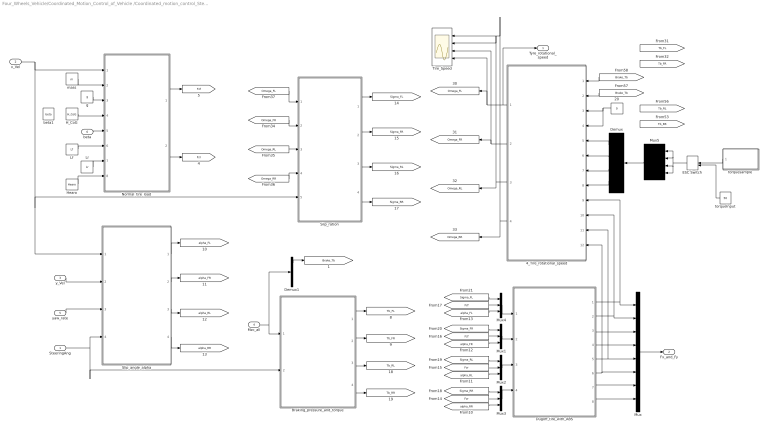
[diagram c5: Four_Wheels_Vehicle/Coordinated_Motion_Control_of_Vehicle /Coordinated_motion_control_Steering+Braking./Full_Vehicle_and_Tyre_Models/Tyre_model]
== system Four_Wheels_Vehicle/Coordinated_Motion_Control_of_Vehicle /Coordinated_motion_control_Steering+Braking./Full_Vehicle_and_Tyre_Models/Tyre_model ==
  SteeringAng : Inport
  x_Vel : Inport  Port=2
  y_Vel : Inport  Port=3
  Mzc_all : Inport  Port=4
  yaw_rate : Inport  Port=5
  beta : Inport  Port=6
  20 : Constant  Value=0
  4_Tire_rotational_speed : Subsystem
  Braking_pressure_and_torque : Subsystem
  Demux : Demux
  Demux1 : Demux
  Dugoff_tire_with_ABS : Subsystem
  ESC Switch : ManualSwitch
  H_CoG : Constant  Value=H_CoG
  Hearo : Constant  Value=Hearo
  Lf : Constant  Value=Lf
  Lr : Constant  Value=Lr
  Mux : Mux  Inputs=8
  Mux{1..4} (4 alike) : Mux  Inputs=3
  Mux5 : Mux
  Normal_tire_load : Subsystem
  Slip_angle_alpha : Subsystem
  Slip_ration : Subsystem
  Tire_Speed : Scope  NumInputPorts=4
  beta1 : Constant  Value=beta
  g : Constant  Value=g
  mass : Constant  Value=m
  torqueInput : Constant  Value=50
  "torquesample " : Subsystem  Tag=STV Subsys  LoadFcn=sigbuilder_block('load');  StartFcn=sigbuilder_block('start');  StopFcn=sigbuilder_block('stop');  ClipboardFcn=sigbuilder_block('clipboard');
  Tyre_rotational_speed : Outport
  Fx_and_Fy : Outport  Port=2
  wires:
  Braking_pressure_and_torque/4(Tb_RR) -> [Tb_RR]
  Braking_pressure_and_torque/1(Tb_FL) -> [Tb_FL]
  Braking_pressure_and_torque/2(Tb_FR) -> [Tb_FR]
  Braking_pressure_and_torque/3(Tb_RL) -> [Tb_RL]
  yaw_rate/1 -> Slip_angle_alpha/3(yaw_rate)
  Slip_ration/4(Sigma_RR) -> [Sigma_RR]
  [alpha_RL] -> Mux2/3
  Mux2/1 -> Dugoff_tire_with_ABS/3(In5)
  y_Vel/1 -> Slip_angle_alpha/2(y_Vel)
  Slip_ration/3(Sigma_RL) -> [Sigma_RL]
  Slip_ration/1(Sigma_FL) -> [Sigma_FL]
  Mux3/1 -> Dugoff_tire_with_ABS/4(In3)
  Mux1/1 -> Dugoff_tire_with_ABS/2(In2)
  Mux4/1 -> Dugoff_tire_with_ABS/1(In1)
  [alpha_RR] -> Mux3/3
  Slip_ration/2(Sigma_FR) -> [Sigma_FR]
  Lr/1 -> Normal_tire_load/7(Lr)
  4_Tire_rotational_speed/1(Omega_FL) -> Tyre_rotational_speed/1, Tire_Speed/4, [Omega_FL]
  Demux/2 -> 4_Tire_rotational_speed/6(Td_FR)
  "torquesample "/1(Signal 1) -> ESC Switch/1
  Dugoff_tire_with_ABS/5(Fx_RL) -> Mux/5, 4_Tire_rotational_speed/11(Fx_RL)
  SteeringAng/1 -> Braking_pressure_and_torque/2(SteeringAng), Slip_angle_alpha/4(Steering_Ang.)
  [Sigma_RL] -> Mux2/1
  Lf/1 -> Normal_tire_load/6(Lf)
  H_CoG/1 -> Normal_tire_load/4(H_CoG)
  4_Tire_rotational_speed/3(Omega_RL) -> Tire_Speed/2, [Omega_RL]
  Mux5/1 -> Demux/1
  ESC Switch/1 -> Mux5/4, Mux5/3, Mux5/1, Mux5/2
  [Omega_FR] -> Slip_ration/2(Omega_FR)
  Demux/3 -> 4_Tire_rotational_speed/7(Td_RL)
  [alpha_FR] -> Mux1/3
  Dugoff_tire_with_ABS/6(Fx_RR) -> Mux/6, 4_Tire_rotational_speed/12(Fx_RR)
  [alpha_FL] -> Mux4/3
  Demux/4 -> 4_Tire_rotational_speed/8(Td_RR)
  [Omega_FL] -> Slip_ration/1(Omega_FL)
  [Omega_RR] -> Slip_ration/4(Omega_RR)
  [Sigma_FR] -> Mux1/1
  x_Vel/1 -> Slip_angle_alpha/1(x_Vel), Slip_ration/5(x_Vel), Normal_tire_load/1(x_Vel)
  [Omega_RL] -> Slip_ration/3(Omega_RL)
  Dugoff_tire_with_ABS/2(Fx_FR) -> Mux/2, 4_Tire_rotational_speed/10(Fx_FR)
  [Sigma_RR] -> Mux3/1
  Dugoff_tire_with_ABS/1(Fx_FL) -> Mux/1, 4_Tire_rotational_speed/9(Fx_FL)
  beta/1 -> Normal_tire_load/5(beta)
  mass/1 -> Normal_tire_load/2(mass)
  [Sigma_FL] -> Mux4/1
  4_Tire_rotational_speed/2(Omega_FR) -> Tire_Speed/3, [Omega_FR]
  Normal_tire_load/2(Fz_r) -> [Fzr]
  Hearo/1 -> Normal_tire_load/8(Hearo)
  g/1 -> Normal_tire_load/3(g)
  Demux/1 -> 4_Tire_rotational_speed/5(Td_FL)
  torqueInput/1 -> ESC Switch/2
  Slip_angle_alpha/4(alpha_RR) -> [alpha_RR]
  [Fzf] -> Mux4/2
  20/1 -> 4_Tire_rotational_speed/4(Tb_RR), 4_Tire_rotational_speed/3(Tb_RL)
  4_Tire_rotational_speed/4(Omega_RR) -> Tire_Speed/1, [Omega_RR]
  [Fzr] -> Mux3/2
  [Brake_Tb] -> 4_Tire_rotational_speed/1(Tb_FL)
  [Brake_Tb] -> 4_Tire_rotational_speed/2(Tb_FR)
  Normal_tire_load/1(Fz_f) -> [Fzf]
  [Fzr] -> Mux2/2
  [Fzf] -> Mux1/2
  Slip_angle_alpha/3(alpha_RL) -> [alpha_RL]
  Slip_angle_alpha/1(alpha_FL) -> [alpha_FL]
  Slip_angle_alpha/2(alpha_FR) -> [alpha_FR]
  Dugoff_tire_with_ABS/8(Fy_RR) -> Mux/8
  Dugoff_tire_with_ABS/7(Fy_RL) -> Mux/7
  Dugoff_tire_with_ABS/4(Fy_FR) -> Mux/4
  Dugoff_tire_with_ABS/3(Fy_FL) -> Mux/3
  Mux/1 -> Fx_and_Fy/1
  Mzc_all/1 -> Demux1/1, Braking_pressure_and_torque/1(Mzc_all)
  Demux1/1 -> [Brake_Tb]

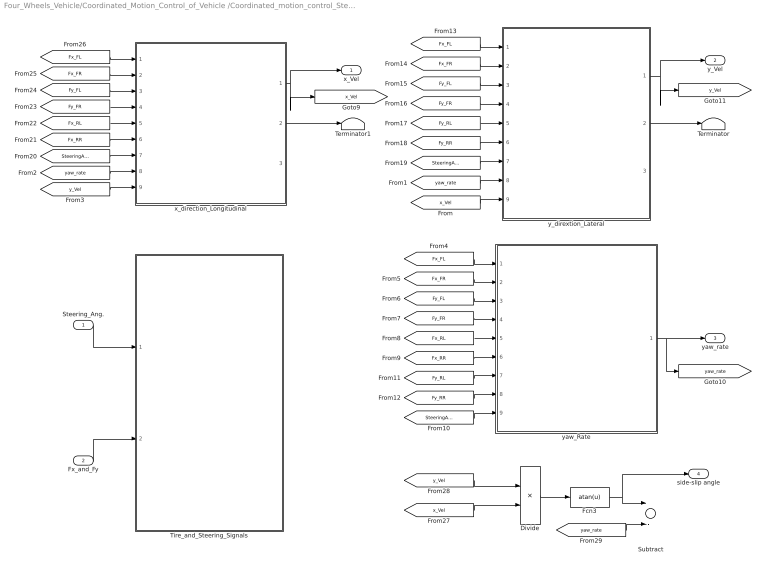
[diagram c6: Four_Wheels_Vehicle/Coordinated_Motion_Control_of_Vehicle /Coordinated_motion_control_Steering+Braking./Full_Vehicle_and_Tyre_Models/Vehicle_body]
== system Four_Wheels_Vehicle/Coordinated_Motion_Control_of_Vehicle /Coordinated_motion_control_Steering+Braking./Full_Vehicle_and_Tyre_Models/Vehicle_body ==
  Steering_Ang. : Inport
  Fx_and_Fy : Inport  Port=2
  Divide : Product  Inputs=*/
  Fcn3 : Fcn  Expr=atan(u)
  Subtract : Sum  Inputs=+-
  Terminator : Terminator
  Terminator1 : Terminator
  Tire_and_Steering_Signals : Subsystem
  x_direction_Longitudinal : Subsystem
  y_dirextion_Lateral : Subsystem
  yaw_Rate : Subsystem
  x_Vel : Outport
  y_Vel : Outport  Port=2
  yaw_rate : Outport  Port=3
  side-slip angle : Outport  Port=4
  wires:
  y_dirextion_Lateral/2(y total force) -> Terminator/1
  x_direction_Longitudinal/2(x total force) -> Terminator1/1
  x_direction_Longitudinal/1(x_Vel) -> [x_Vel], x_Vel/1
  [x_Vel] -> y_dirextion_Lateral/9(x_Vel)
  [yaw_rate] -> y_dirextion_Lateral/8(yaw_rate)
  [yaw_rate] -> x_direction_Longitudinal/8(yaw_rate)
  y_dirextion_Lateral/1(y_Vel) -> [y_Vel], y_Vel/1
  [y_Vel] -> x_direction_Longitudinal/9(y_Vel)
  [Fx_FL] -> yaw_Rate/1(Fx_FL)
  [Fx_FR] -> yaw_Rate/2(Fx_FR)
  [Fy_FL] -> yaw_Rate/3(Fy_FL)
  [Fy_FR] -> yaw_Rate/4(Fy_FR)
  [Fx_RL] -> yaw_Rate/5(Fx_RL)
  [Fx_RR] -> yaw_Rate/6(Fx_RR)
  [Fy_RL] -> yaw_Rate/7(Fy_RL)
  [Fy_RR] -> yaw_Rate/8(Fy_RR)
  [SteeringAng] -> yaw_Rate/9(Steering_Ang.)
  [Fx_FL] -> y_dirextion_Lateral/1(Fx_FL)
  [Fx_FR] -> y_dirextion_Lateral/2(Fx_FR)
  [Fy_FL] -> y_dirextion_Lateral/3(Fy_FL)
  [Fy_FR] -> y_dirextion_Lateral/4(Fy_FR)
  [Fy_RL] -> y_dirextion_Lateral/5(Fy_RL)
  [Fy_RR] -> y_dirextion_Lateral/6(Fy_RR)
  [SteeringAng] -> y_dirextion_Lateral/7(Steering_Ang.)
  [SteeringAng] -> x_direction_Longitudinal/7(Steering_Ang.)
  [Fx_RR] -> x_direction_Longitudinal/6(Fx_RR)
  [Fx_RL] -> x_direction_Longitudinal/5(Fx_RL)
  [Fy_FR] -> x_direction_Longitudinal/4(Fy_FR)
  [Fy_FL] -> x_direction_Longitudinal/3(Fy_FL)
  [Fx_FR] -> x_direction_Longitudinal/2(Fx_FR)
  [Fx_FL] -> x_direction_Longitudinal/1(Fx_FL)
  yaw_Rate/1(yaw_rate) -> [yaw_rate], yaw_rate/1
  Steering_Ang./1 -> Tire_and_Steering_Signals/1(Steering_Ang.)
  Divide/1 -> Fcn3/1
  Fcn3/1 -> side-slip angle/1, Subtract/1
  [x_Vel] -> Divide/2
  [y_Vel] -> Divide/1
  [yaw_rate] -> Subtract/2
  Fx_and_Fy/1 -> Tire_and_Steering_Signals/2(Fx_and_Fy)

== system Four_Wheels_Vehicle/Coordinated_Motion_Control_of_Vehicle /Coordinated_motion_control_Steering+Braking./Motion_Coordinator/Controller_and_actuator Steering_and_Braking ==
  StteringAng : Inport
  Reference_Steering : Inport  Port=2
  Reference_Sideslip : Inport  Port=3
  Feedback_Steering : Inport  Port=4
  Feedback_Sideslip : Inport  Port=5
  Brake_controller_1 : Subsystem
  Brake_controller_2 : Subsystem
  Brake_controller_3 : Subsystem
  Brake_controller_4 : Subsystem
  Steering_controller : Subsystem
  f : Outport
  Mzc_1 : Outport  Port=2
  Mzc_2 : Outport  Port=3
  Mzc_3 : Outport  Port=4
  Mzc_4 : Outport  Port=5
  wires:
  StteringAng/1 -> Steering_controller/1(StteringAng)
  Reference_Steering/1 -> Steering_controller/2(Reference_Steering)
  Feedback_Steering/1 -> Steering_controller/3(Feedback_Steering)
  Steering_controller/1(f) -> f/1
  Reference_Sideslip/1 -> Brake_controller_4/1(Reference_Sideslip_4), Brake_controller_3/1(Reference_Sideslip_3), Brake_controller_2/1(Reference_Sideslip_2), Brake_controller_1/1(Reference_Sideslip_1)
  Feedback_Sideslip/1 -> Brake_controller_4/2(Feedback_Sideslip_4), Brake_controller_3/2(Feedback_Sideslip_3), Brake_controller_2/2(Feedback_Sideslip_2), Brake_controller_1/2(Feedback_Sideslip_1)
  Brake_controller_1/1(Mzc_1) -> Mzc_1/1
  Brake_controller_2/1(Mzc_2) -> Mzc_2/1
  Brake_controller_3/1(Mzc_3) -> Mzc_3/1
  Brake_controller_4/1(Mzc_4) -> Mzc_4/1

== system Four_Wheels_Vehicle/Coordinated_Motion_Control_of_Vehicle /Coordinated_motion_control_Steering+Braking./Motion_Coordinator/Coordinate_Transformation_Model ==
  note: vehicle heading
  delta_steer (rad) : Inport
  v_x (m/s) : Inport  Port=2
  1/L : Gain  Gain=1/L
  Beta : Scope
  Beta1 : Scope
  Divide : Product  Inputs=*/
  Gain : Gain  Gain=L/2
  Gain1 : Gain  Gain=0.1
  Gain2 : Gain  Gain=0.1
  Gain4 : Gain  Gain=0.345
  Ground : Ground
  Integrator : Integrator
  Integrator1 : Integrator  LimitOutput=on  UpperSaturationLimit=0
  Integrator2 : Integrator
  Product{,1,3..4} (4 alike) : Product
  Sideslip_angle : Scope
  Subtract : Sum  Inputs=+-
  Sum : Sum  Inputs=|+-
  Sum1 : Sum  Inputs=|++
  Terminator : Terminator
  Trigonometric Function : Trigonometry  Operator=cos
  Trigonometric Function1 : Trigonometry
  Trigonometric Function2 : Trigonometry  Operator=atan
  Trigonometric Function3 : Trigonometry  Operator=tan
  steerVsYawrate1 : Scope  NumInputPorts=3
  steerVsYawrate2 : Scope  NumInputPorts=3
  yaw_rate : Product
  X-position : Outport
  Y-position : Outport  Port=2
  yaw_Rate : Outport  Port=3
  Sideslip_beta : Outport  Port=4
  yaw_position : Outport  Port=5
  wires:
  Product/1 -> Sum1/1
  Product1/1 -> Sum/1
  Trigonometric Function/1 -> Product1/2, Product4/2  "cos(psi)"
  Trigonometric Function1/1 -> Product/2, Product3/2  "sin(psi)"
  Integrator2/1 -> Gain1/1  "yaw_heading (rad)"
  Integrator/1 -> steerVsYawrate1/1, X-position/1
  Integrator1/1 -> steerVsYawrate1/2, Y-position/1
  v_x (m/s)/1 -> Product/1, Product1/1, 1/L/1  "v_x (m/s)"
  yaw_rate/1 -> steerVsYawrate2/1, Gain/1, yaw_Rate/1, Beta1/1, Subtract/2, Gain2/1
  1/L/1 -> yaw_rate/1  "v_x / L"
  Sum/1 -> steerVsYawrate2/2, Integrator/1, Divide/2  "v_X (m/s)"
  Sum1/1 -> Gain4/1  "v_Y (m/s)"
  Gain/1 -> Product3/1, Product4/1  "L/2*psi-dot"
  Product3/1 -> Sum/2
  Product4/1 -> Sum1/2
  Ground/1 -> Trigonometric Function3/1
  Trigonometric Function3/1 -> Terminator/1
  Divide/1 -> Trigonometric Function2/1
  delta_steer (rad)/1 -> yaw_rate/2
  Gain1/1 -> Trigonometric Function/1, steerVsYawrate1/3, yaw_position/1, Trigonometric Function1/1
  Gain2/1 -> Integrator2/1
  Trigonometric Function2/1 -> Sideslip_angle/1, Sideslip_beta/1, Subtract/1
  Gain4/1 -> steerVsYawrate2/3, Integrator1/1, Divide/1
  Subtract/1 -> Beta/1

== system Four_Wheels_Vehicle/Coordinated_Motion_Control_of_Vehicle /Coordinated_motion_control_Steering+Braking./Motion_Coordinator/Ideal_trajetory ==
  SteeringAng : Inport
  Constant_speed (m/s)1 : Constant  Value=4.55
  Coordinate_Transformation_Model : Subsystem
  Gain4 : Gain  Gain=10
  Y-position : Outport
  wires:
  Coordinate_Transformation_Model/2(Y-position) -> Y-position/1
  Gain4/1 -> Coordinate_Transformation_Model/1(delta_steer (rad))
  Constant_speed (m/s)1/1 -> Coordinate_Transformation_Model/2(v_x (m/s))
  SteeringAng/1 -> Gain4/1

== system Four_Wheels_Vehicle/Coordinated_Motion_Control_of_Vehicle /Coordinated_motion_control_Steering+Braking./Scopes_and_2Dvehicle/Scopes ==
  SteeringAng : Inport
  x_Vel : Inport  Port=2
  y_Vel : Inport  Port=3
  yaw_rate : Inport  Port=4
  sideslipAng : Inport  Port=5
  Ideal : Inport  Port=6
  Integrator : Integrator  LimitOutput=on
  Integrator1 : Integrator  LimitOutput=on  UpperSaturationLimit=0
  Trajectory_Comparison : Scope  NumInputPorts=2
  steerVsYawrate : Scope  NumInputPorts=2
  x_y_directions : Scope  NumInputPorts=2
  x_y_yaw : Scope  NumInputPorts=4
  Ideal_trajectory : Outport
  Estimated_trajectory : Outport  Port=2
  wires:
  Integrator/1 -> x_y_directions/1
  x_Vel/1 -> Integrator/1, x_y_yaw/1
  y_Vel/1 -> Integrator1/1, x_y_yaw/2
  Ideal/1 -> Trajectory_Comparison/1, Ideal_trajectory/1
  Integrator1/1 -> x_y_directions/2, Estimated_trajectory/1, Trajectory_Comparison/2
  yaw_rate/1 -> steerVsYawrate/2, x_y_yaw/3
  sideslipAng/1 -> x_y_yaw/4
  SteeringAng/1 -> steerVsYawrate/1

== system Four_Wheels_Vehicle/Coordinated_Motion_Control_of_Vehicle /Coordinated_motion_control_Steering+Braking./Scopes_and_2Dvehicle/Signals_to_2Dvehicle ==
  SteeringAng. : Inport
  x_Vel. : Inport  Port=2
  y_Vel. : Inport  Port=3
  yaw_rate. : Inport  Port=4
  Ideal. : Inport  Port=5
  Gain3 : Gain  Gain=0.05
  Integrator2 : Integrator  LimitOutput=on
  Integrator3 : Integrator  LimitOutput=on  UpperSaturationLimit=0
  Integrator4 : Integrator  LimitOutput=on  UpperSaturationLimit=0
  x_Vel : Outport
  y_Vel : Outport  Port=2
  yaw_rate : Outport  Port=3
  SteeringAng : Outport  Port=4
  Ideal : Outport  Port=5
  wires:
  x_Vel./1 -> Integrator2/1
  y_Vel./1 -> Integrator3/1
  Integrator4/1 -> Gain3/1
  yaw_rate./1 -> Integrator4/1
  Integrator2/1 -> x_Vel/1
  Integrator3/1 -> y_Vel/1
  Gain3/1 -> yaw_rate/1
  SteeringAng./1 -> SteeringAng/1
  Ideal./1 -> Ideal/1

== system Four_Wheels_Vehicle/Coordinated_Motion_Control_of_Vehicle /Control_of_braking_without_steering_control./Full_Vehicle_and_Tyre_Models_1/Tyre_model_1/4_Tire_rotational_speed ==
  Tb_FL_1 : Inport
  Tb_FR_1 : Inport  Port=2
  Tb_RL_1 : Inport  Port=3
  Tb_RR_1 : Inport  Port=4
  Td_FL_1 : Inport  Port=5
  Td_FR_1 : Inport  Port=6
  Td_RL_1 : Inport  Port=7
  Td_RR_1 : Inport  Port=8
  Fx_FL_1 : Inport  Port=9
  Fx_FR_1 : Inport  Port=10
  Fx_RL_1 : Inport  Port=11
  Fx_RR_1 : Inport  Port=12
  Tire_speed_FL : Subsystem
  Tire_speed_FR : Subsystem
  Tire_speed_RL : Subsystem
  Tire_speed_RR : Subsystem
  Omega_FL_1 : Outport
  Omega_FR_1 : Outport  Port=2
  Omega_RL_1 : Outport  Port=3
  Omega_RR_1 : Outport  Port=4
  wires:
  Td_RR_1/1 -> Tire_speed_RR/2(Td_RR_1)
  Td_RL_1/1 -> Tire_speed_RL/2(Td_RL_1)
  Tire_speed_RR/1(Omega_RR_1) -> Omega_RR_1/1
  Fx_RR_1/1 -> Tire_speed_RR/3(Fx_RR_1)
  Tb_RR_1/1 -> Tire_speed_RR/1(Tb_RR_1)
  Tire_speed_RL/1(Omega_RL_1) -> Omega_RL_1/1
  Fx_RL_1/1 -> Tire_speed_RL/3(Fx_RL_1)
  Tb_RL_1/1 -> Tire_speed_RL/1(Tb_RL_1)
  Tire_speed_FR/1(Omega_FR_1) -> Omega_FR_1/1
  Fx_FR_1/1 -> Tire_speed_FR/3(Fx_FR_1)
  Td_FR_1/1 -> Tire_speed_FR/2(Td_FR_1)
  Tb_FR_1/1 -> Tire_speed_FR/1(Tb_FR_1)
  Tire_speed_FL/1(Omega_FL_1) -> Omega_FL_1/1
  Fx_FL_1/1 -> Tire_speed_FL/3(Fx_FL_1)
  Td_FL_1/1 -> Tire_speed_FL/2(Td_FL_1)
  Tb_FL_1/1 -> Tire_speed_FL/1(Tb_FL_1)

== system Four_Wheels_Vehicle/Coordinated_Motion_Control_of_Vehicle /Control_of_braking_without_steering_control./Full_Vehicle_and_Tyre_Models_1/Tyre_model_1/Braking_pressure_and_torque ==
  Mzc_all_1 : Inport
  SteeringAng : Inport  Port=2
  Braking_pressure_and_torque_FL : MATLAB Function  TreatAsAtomicUnit=on
  Braking_pressure_and_torque_FR : MATLAB Function  TreatAsAtomicUnit=on
  Braking_pressure_and_torque_RL : MATLAB Function  TreatAsAtomicUnit=on
  Braking_pressure_and_torque_RR : MATLAB Function  TreatAsAtomicUnit=on
  Demux : Demux
  reff{,1..3} (4 alike) : Constant  Value=reff
  tw{,1..3} (4 alike) : Constant  Value=1.65
  Tb_FL_1 : Outport
  Tb_FR_1 : Outport  Port=2
  Tb_RL_1 : Outport  Port=3
  Tb_RR_1 : Outport  Port=4
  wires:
  Demux/4 -> Braking_pressure_and_torque_RR/1(M)
  Demux/3 -> Braking_pressure_and_torque_RL/1(M)
  Demux/2 -> Braking_pressure_and_torque_FR/1(M)
  Demux/1 -> Braking_pressure_and_torque_FL/1(M)
  Mzc_all_1/1 -> Demux/1
  SteeringAng/1 -> Braking_pressure_and_torque_FL/4(SteeringAng), Braking_pressure_and_torque_FR/4(SteeringAng)
  tw/1 -> Braking_pressure_and_torque_FL/3(tw)
  Braking_pressure_and_torque_RL/2(Tb_RL) -> Tb_RL_1/1
  reff2/1 -> Braking_pressure_and_torque_RL/2(reff)
  tw1/1 -> Braking_pressure_and_torque_FR/3(tw)
  tw3/1 -> Braking_pressure_and_torque_RR/3(tw)
  Braking_pressure_and_torque_FL/2(Tb_FL) -> Tb_FL_1/1
  reff/1 -> Braking_pressure_and_torque_FL/2(reff)
  Braking_pressure_and_torque_RR/2(Tb_RR) -> Tb_RR_1/1
  tw2/1 -> Braking_pressure_and_torque_RL/3(tw)
  reff3/1 -> Braking_pressure_and_torque_RR/2(reff)
  reff1/1 -> Braking_pressure_and_torque_FR/2(reff)
  Braking_pressure_and_torque_FR/2(Tb_FR) -> Tb_FR_1/1
